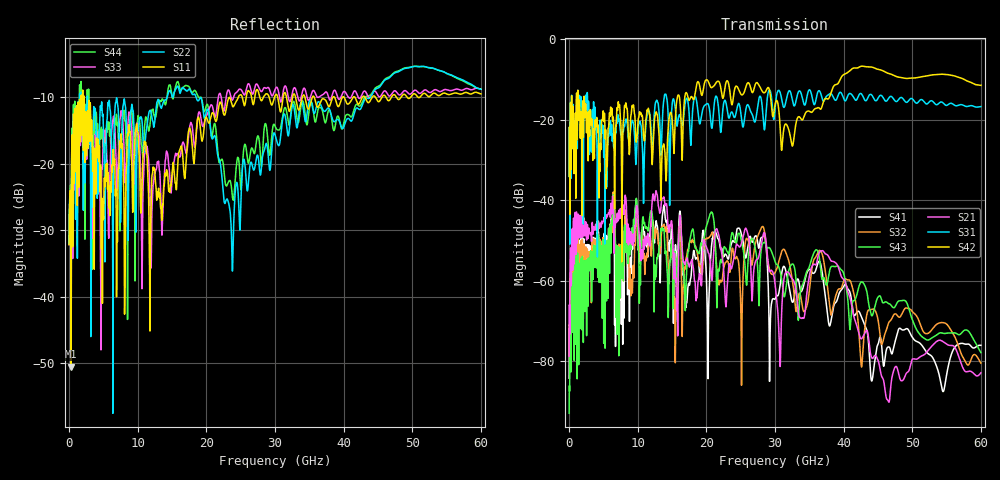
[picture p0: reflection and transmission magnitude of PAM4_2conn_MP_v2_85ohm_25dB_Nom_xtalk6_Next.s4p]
! Info: Touchstone file created by Circ.  Input file=FAB50GbE_2conn_Midplane_Examax_Topo2_v2_85ohm_25dB_Nom.circ
# Hz S RI R 50
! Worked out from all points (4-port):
!   6000 points, 10 MHz to 60 GHz, reference 50 ohm
!   strongest paths, dB at 10 MHz, 15.01 GHz, 30.01 GHz, 45.01 GHz, 60 GHz:
!     S42: -34.0, -19.7, -16.3, -7.5, -11.4
!     S31: -34.1, -16.3, -17.2, -14.7, -16.7
!     S21: -78.8, -46.2, -60.8, -79.7, -82.9
!     S43: -93.0, -50.8, -55.3, -64.1, -77.9
!     S32: -78.5, -51.5, -58.0, -69.7, -80.5
!     S41: -84.2, -47.3, -64.6, -75.8, -76.1
!   lowest |S11| = -50.5 dB at 310 MHz (marker M1), VSWR 1.01, Z = 50.2 + j0.238 ohm
!   |S11| at or under -10 dB: start of sweep to 1.747 GHz; 2.202 GHz to 24.67 GHz (22.46 GHz wide, 167 % of centre); 35.71 GHz to 38.47 GHz (2.763 GHz wide, 7.45 % of centre)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
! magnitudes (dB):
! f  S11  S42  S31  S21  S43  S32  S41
! 10 MHz  -32.2  -34.0  -34.1  -78.8  -93.0  -78.5  -84.2
! 310 MHz  -50.5  -21.5  -22.4  -61.3  -67.6  -73.2  -65.9
! 6.43 GHz  -18.0  -19.3  -24.7  -41.2  -38.7  -38.0  -45.8
! 12.53 GHz  -21.9  -19.1  -16.4  -39.4  -58.3  -49.4  -48.3
! 15.52 GHz  -23.0  -18.8  -17.8  -59.8  -53.9  -72.9  -51.2
! 20.73 GHz  -12.7  -12.0  -21.7  -58.4  -42.9  -48.4  -51.9
! 60 GHz  -9.5  -11.4  -16.7  -82.9  -77.9  -80.5  -76.1
